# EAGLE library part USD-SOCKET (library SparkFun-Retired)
microSD Socket Push-push type uSD socket. Schematic element and footprint production proven. Spark Fun Electronics SKU : PRT-00127. tDoc lines correctly indicate media card edge positions when inserting (unlocked, locked, depressed). NOTE: CD1 and CD2 are connected internally
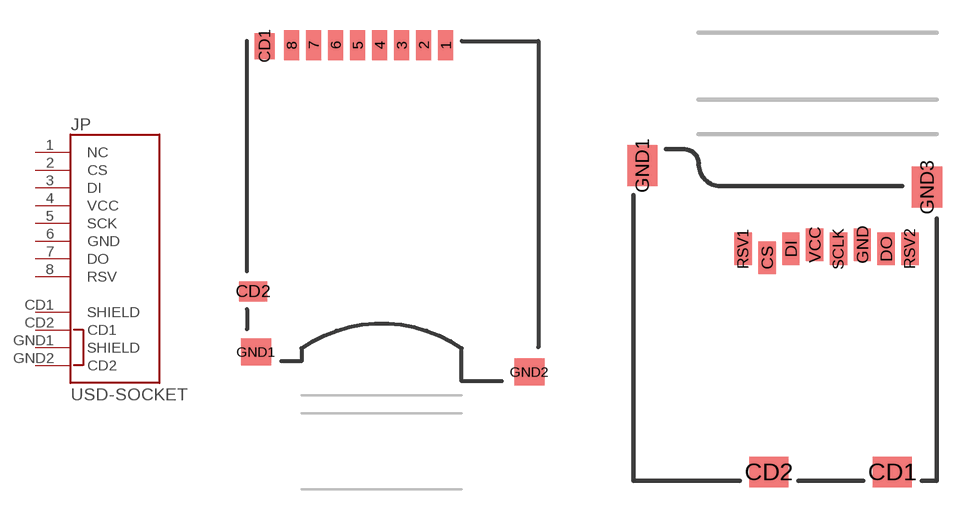
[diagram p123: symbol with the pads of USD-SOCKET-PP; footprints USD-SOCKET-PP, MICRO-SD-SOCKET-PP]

Designator prefix JP

## USD-SOCKETUSD  [USD-SOCKET-PP]
1  NC
2  CS
3  DI
4  VCC
5  SCK
6  GND
7  DO
8  RSV
CD1  SHIELD
CD2  CD1
GND1  SHIELD
GND2  CD2

## USD-SOCKETNEW (PROD_ID: CONN-07820)  [MICRO-SD-SOCKET-PP]
CD1  CD1
CD2  CD2
CS  CS
DI  DI
DO  DO
GND  GND
GND1  SHIELD
GND3  SHIELD
RSV1  NC
RSV2  RSV
SCLK  SCK
VCC  VCC

## USD-SOCKET (PROD_ID: CONN-07820)  [MICROSD_1:1]
1  NC
2  CS
3  DI
4  VCC
5  SCK
6  GND
7  DO
8  RSV
CD1  CD1
CD2  CD2
GND1  SHIELD
GND3  SHIELD

## Footprint USD-SOCKET-PP (pad centres in mm)
OLD Production Socket. DO NOT USE for production boards.
smd 0.75 x 1.5: 1 3.2,16.8; 2 2.1,16.8; 3 1,16.8; 4 -0.1,16.8; 5 -1.2,16.8; 6 -2.3,16.8; 7 -3.4,16.8; 8 -4.5,16.8
smd 1 x 1.3: CD1 -5.85,16.75
smd 1.4 x 1: CD2 -6.425,4.5
smd 1.5 x 1.35: GND1 -6.275,1.475; GND2 7.375,0.475

## Footprint MICRO-SD-SOCKET-PP (pad centres in mm)
smd 1.8 x 1.4: CD1 -2.05,0.4; CD2 -7.75,0.4
smd 0.8 x 1.5: CS -7.84,10.3; DI -6.74,10.7; DO -2.34,10.7; GND -3.44,10.9; RSV1 -8.94,10.7; RSV2 -1.24,10.7; SCLK -4.54,10.7; VCC -5.64,10.9
smd 1.4 x 1.9: GND1 -13.6,14.55; GND3 -0.45,13.55

## Footprint MICROSD_1:1 (pad centres in mm)
smd 0.8 x 1.5: 1 5.096,10.919; 2 6.218,10.519; 3 7.274,10.853; 4 8.367,10.982; 5 9.421,10.828; 6 10.539,10.973; 7 11.648,10.819; 8 12.721,10.819
smd 1.8 x 1.4: CD1 11.92,0.4; CD2 6.22,0.4
smd 1.4 x 1.9: GND1 0.497,14.55; GND3 13.52,13.55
